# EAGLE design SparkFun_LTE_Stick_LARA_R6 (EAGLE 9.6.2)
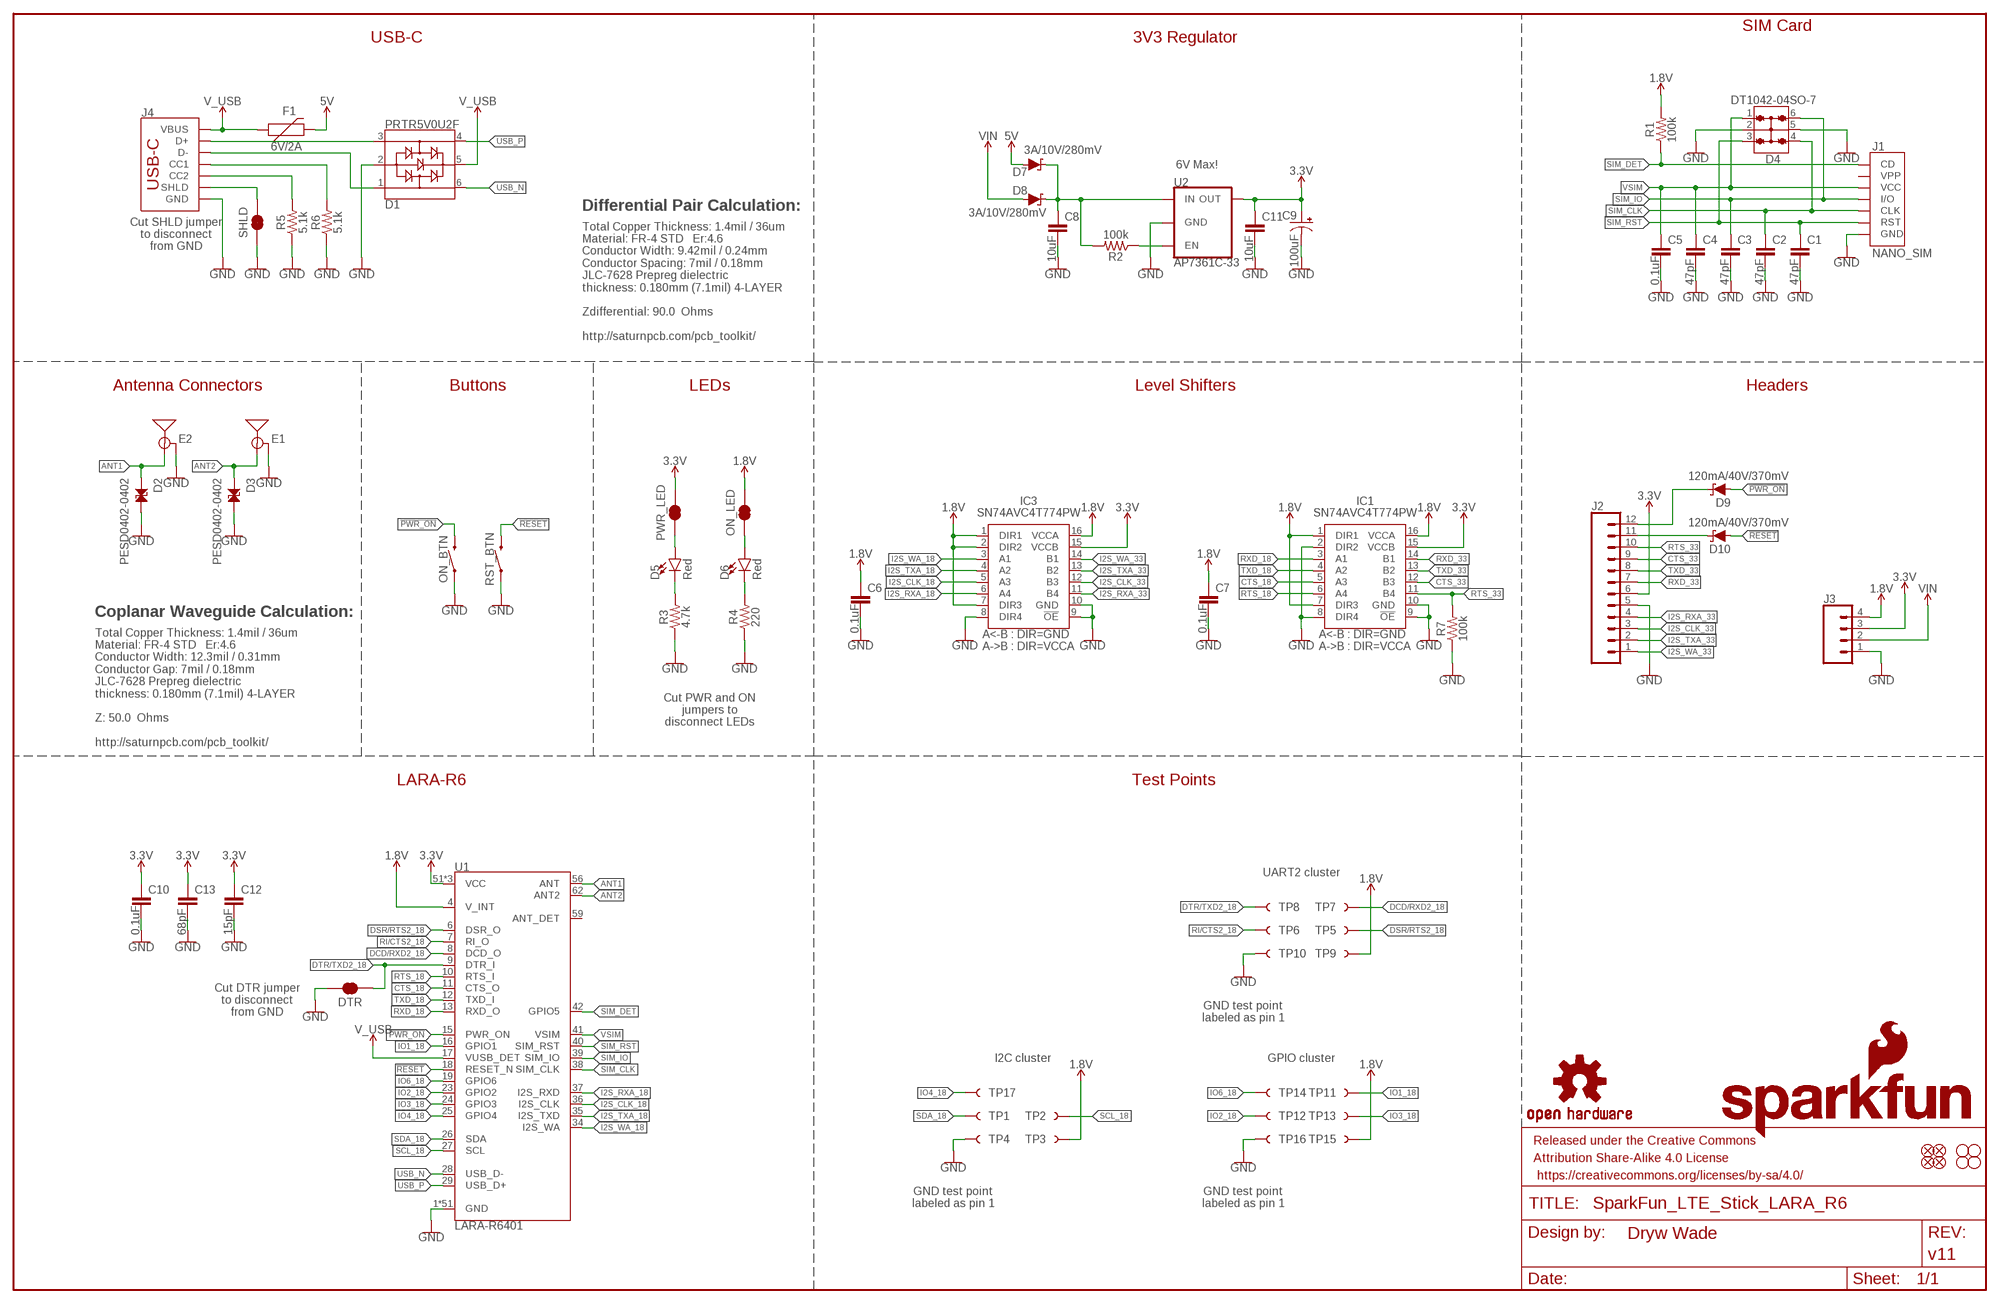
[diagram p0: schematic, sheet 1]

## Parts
C1  47pF  47PF-0603-50V-5%  [0603]
C2  47pF  47PF-0603-50V-5%  [0603]
C3  47pF  47PF-0603-50V-5%  [0603]
C4  47pF  47PF-0603-50V-5%  [0603]
C5  0.1uF  0.1UF-0603-25V-5%  [0603]
C6  0.1uF  0.1UF-0603-25V-5%  [0603]
C7  0.1uF  0.1UF-0603-25V-5%  [0603]
C8  10uF  10UF-0805-25V-10%  [0805]
C9  100uF  100UF-POLAR-25V-20%(ELEC)  [PANASONIC_D]
C10  0.1uF  0.1UF-0603-25V-5%  [0603]
C11  10uF  10UF-0805-25V-10%  [0805]
C12  15pF  15PF-0603-50V-5%  [0603]
C13  68pF  68PF-0603-50V-5%  [0603]
D1  PRTR5V0U2F  [SOT886]
D2  PESD0402-0402  [0402]
D3  PESD0402-0402  [0402]
D4  DT1042-04SO-7  TVS_DIODE_ARRAY_4_ESDA6V1BC6  [SOT23-6L]
D5  Red  LED-RED_0603-KB  [LED-0603]
D6  Red  LED-RED_0603-KB  [LED-0603]
D7  3A/10V/280mV  DIODE-SCHOTTKY-BAT60A  [SOD-323]
D8  3A/10V/280mV  DIODE-SCHOTTKY-BAT60A  [SOD-323]
D9  120mA/40V/370mV  DIODE-SCHOTTKY-RB751S40  [SOD-523]
D10  120mA/40V/370mV  DIODE-SCHOTTKY-RB751S40  [SOD-523]
DTR  JUMPER-SMT_2_NC_TRACE_SILK  [SMT-JUMPER_2_NC_TRACE_SILK]
E1  ANTENNA-SMA-GROUNDEDEDGE_SMA  [SMA-EDGE]
E2  ANTENNA-SMA-GROUNDEDEDGE_SMA  [SMA-EDGE]
F1  6V/2A  PPTC_6V2A  [1210]
FD1  FIDUCIAL1X2  [FIDUCIAL-1X2]
FD2  FIDUCIAL1X2  [FIDUCIAL-1X2]
FD3  FIDUCIAL1X2  [FIDUCIAL-1X2]
FD4  FIDUCIAL1X2  [FIDUCIAL-1X2]
FRAME1  FRAME-LEDGER  [CREATIVE_COMMONS]
H1  STAND-OFF  [STAND-OFF]
H2  STAND-OFF  [STAND-OFF]
H3  STAND-OFF  [STAND-OFF]
H4  STAND-OFF  [STAND-OFF]
IC1  SN74AVC4T774PW  [SOP65P640X120-16N]
IC3  SN74AVC4T774PW  [SOP65P640X120-16N]
J1  NANO_SIM  SIMHOLDER_WITH_CD-PUSHPUSH  [NANO_SIM_PP]
J2  CONN_12NO_SILK  [1X12_NO_SILK]
J3  CONN_041X04_NO_SILK_NO_POP  [1X04_NO_SILK]
J4  USB_C_4-LAYER_PADS  [USB-C-16P_4LAYER-PADS]
LOGO1  SFE_LOGO_NAME_FLAME.1_INCH  [SFE_LOGO_NAME_FLAME_.1]
LOGO2  OSHW-LOGOM  [OSHW-LOGO-M]
ON_BTN  MOMENTARY-SWITCH-SPST-SMD-4.6X2.8MM  [TACTILE_SWITCH_SMD_4.6X2.8MM]
ON_LED  JUMPER-SMT_2_NC_TRACE_SILK  [SMT-JUMPER_2_NC_TRACE_SILK]
PWR_LED  JUMPER-SMT_2_NC_TRACE_SILK  [SMT-JUMPER_2_NC_TRACE_SILK]
R1  100k  100KOHM-0603-1/10W-1%  [0603]
R2  100k  100KOHM-0603-1/10W-1%  [0603]
R3  4.7k  4.7KOHM-0603-1/10W-1%  [0603]
R4  220  220OHM-0603-1/10W-1%  [0603]
R5  5.1k  5.1KOHM5.1KOHM-0603-1/10W-1%  [0603]
R6  5.1k  5.1KOHM5.1KOHM-0603-1/10W-1%  [0603]
R7  100k  100KOHM-0603-1/10W-1%  [0603]
RST_BTN  MOMENTARY-SWITCH-SPST-SMD-4.6X2.8MM  [TACTILE_SWITCH_SMD_4.6X2.8MM]
SHLD  JUMPER-SMT_2_NC_TRACE_SILK  [SMT-JUMPER_2_NC_TRACE_SILK]
TP1  TEST-POINT3X5  [PAD.03X.05]
TP2  TEST-POINT3X5  [PAD.03X.05]
TP3  TEST-POINT3X5  [PAD.03X.05]
TP4  TEST-POINT3X5  [PAD.03X.05]
TP5  TEST-POINT3X5  [PAD.03X.05]
TP6  TEST-POINT3X5  [PAD.03X.05]
TP7  TEST-POINT3X5  [PAD.03X.05]
TP8  TEST-POINT3X5  [PAD.03X.05]
TP9  TEST-POINT3X5  [PAD.03X.05]
TP10  TEST-POINT3X5  [PAD.03X.05]
TP11  TEST-POINT3X5  [PAD.03X.05]
TP12  TEST-POINT3X5  [PAD.03X.05]
TP13  TEST-POINT3X5  [PAD.03X.05]
TP14  TEST-POINT3X5  [PAD.03X.05]
TP15  TEST-POINT3X5  [PAD.03X.05]
TP16  TEST-POINT3X5  [PAD.03X.05]
TP17  TEST-POINT3X5  [PAD.03X.05]
U1  LARA-R6401  LARA-R6_R6401_USA  [LARA-LGA]
U2  AP7361C-33  AP7361C-33FGEUDFN-8  [UDFN-8]

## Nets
1.8V: C6.1 C7.1 IC1.1(DIR1) IC1.7(DIR3) IC1.16(VCCA) IC3.1(DIR1) IC3.2(DIR2) IC3.7(DIR3) IC3.16(VCCA) J3.4 ON_LED.2 R1.2 TP3.1 TP9.1 TP15.1 U1.4(V_INT)
3.3V: C9.+ C10.1 C11.1 C12.1 C13.1 IC1.15(VCCB) IC3.15(VCCB) J2.6 J3.3 PWR_LED.2 U1.51(VCC) U1.52(VCC) U1.53(VCC) U2.1(OUT)
5V: D7.A F1.2
!PWR_ON!: D9.A ON_BTN.3 ON_BTN.4 U1.15(PWR_ON)
!RESET!: D10.A RST_BTN.3 RST_BTN.4 U1.18(RESET_N)
ANT1 [RF]: D2.1 E2.SIG(SIGNAL) U1.56(ANT)
ANT2 [RF]: D3.1 E1.SIG(SIGNAL) U1.62(ANT2)
CTS_18: IC1.5(A3) U1.11(CTS_O)
CTS_33: IC1.12(B3) J2.9
DCD/RXD2_18: TP7.1 U1.8(DCD_O)
DSR/RTS2_18: TP5.1 U1.6(DSR_O)
DTR/TXD2_18: DTR.2 TP8.1 U1.9(DTR_I)
EN: R2.1 U2.5(EN)
GND: C1.2 C2.2 C3.2 C4.2 C5.2 C6.2 C7.2 C8.2 C9.- C10.2 C11.2 C12.2 C13.2 D1.2 D2.2 D3.2 D4.2 D4.5 DTR.1 E1.GND@0(GND) E1.GND@1(GND) E1.GND@2(GND) E1.GND@3(GND) E2.GND@0(GND) E2.GND@1(GND) E2.GND@2(GND) E2.GND@3(GND) IC1.2(DIR2) IC1.8(DIR4) IC1.9(!OE) IC1.10(GND) IC3.8(DIR4) IC3.9(!OE) IC3.10(GND) J1.A1(GND) J1.A2(GND) J1.A3(GND) J1.A4(GND) J1.C5(GND) J2.5 J3.1 J4.GND J4.GND2(GND) ON_BTN.1 ON_BTN.2 R3.1 R4.1 R5.1 R6.1 R7.1 RST_BTN.1 RST_BTN.2 SHLD.1 TP4.1 TP10.1 TP16.1 U1.1(GND) U1.3(GND) U1.5(GND) U1.14(GND) U1.20(GND) U1.21(GND) U1.22(GND) U1.30(GND) U1.32(GND) U1.43(GND) U1.50(GND) U1.54(GND) U1.55(GND) U1.57(GND) U1.58(GND) U1.60(GND) U1.61(GND) U1.63(GND) U1.64(GND) U1.65(GND) U1.66(GND) U1.67(GND) U1.68(GND) U1.69(GND) U1.70(GND) U1.71(GND) U1.72(GND) U1.73(GND) U1.74(GND) U1.75(GND) U1.76(GND) U1.77(GND) U1.78(GND) U1.79(GND) U1.80(GND) U1.81(GND) U1.82(GND) U1.83(GND) U1.84(GND) U1.85(GND) U1.86(GND) U1.87(GND) U1.88(GND) U1.89(GND) U1.90(GND) U1.91(GND) U1.92(GND) U1.93(GND) U1.94(GND) U1.95(GND) U1.96(GND) U2.4(GND) U2.EP(GND)
I2S_CLK_18: IC3.5(A3) U1.36(I2S_CLK)
I2S_CLK_33: IC3.12(B3) J2.3
I2S_RXA_18: IC3.6(A4) U1.37(I2S_RXD)
I2S_RXA_33: IC3.11(B4) J2.4
I2S_TXA_18: IC3.4(A2) U1.35(I2S_TXD)
I2S_TXA_33: IC3.13(B2) J2.2
I2S_WA_18: IC3.3(A1) U1.34(I2S_WA)
I2S_WA_33: IC3.14(B1) J2.1
IO1_18: TP11.1 U1.16(GPIO1)
IO2_18: TP12.1 U1.23(GPIO2)
IO3_18: TP13.1 U1.24(GPIO3)
IO4_18: TP17.1 U1.25(GPIO4)
IO6_18: TP14.1 U1.19(GPIO6)
N$1: D5.C R3.2
N$2: D5.A PWR_LED.1
N$3: D6.A ON_LED.1
N$4: D6.C R4.2
N$5: D10.C J2.11
N$6: D9.C J2.12
N$7: C8.1 D7.C D8.C R2.2 U2.8(IN)
N$8: J4.B5(CC2) R5.2
N$9: J4.A5(CC1) R6.2
N$10: D1.3 J4.A6(D+) J4.B6(D+)
N$11: D1.1 J4.A7(D-) J4.B7(D-)
RI/CTS2_18: TP6.1 U1.7(RI_O)
RTS_18: IC1.6(A4) U1.10(RTS_I)
RTS_33: IC1.11(B4) J2.10 R7.2
RXD_18: IC1.3(A1) U1.13(RXD_O)
RXD_33: IC1.14(B1) J2.7
SCL_18: TP2.1 U1.27(SCL)
SDA_18: TP1.1 U1.26(SDA)
SHLD: J4.SHLD1(SHLD) J4.SHLD2(SHLD) J4.SHLD3(SHLD) J4.SHLD4(SHLD) SHLD.2
SIM_CLK: C2.1 D4.4 J1.C3(CLK) U1.38(SIM_CLK)
SIM_DET: J1.CD R1.1 U1.42(GPIO5)
SIM_IO: C3.1 D4.6 J1.C7(I/O) U1.39(SIM_IO)
SIM_RST: C1.1 D4.3 J1.C2(RST) U1.40(SIM_RST)
TXD_18: IC1.4(A2) U1.12(TXD_I)
TXD_33: IC1.13(B2) J2.8
USB_N [USB]: D1.6 U1.28(USB_D-)
USB_P [USB]: D1.4 U1.29(USB_D+)
V_USB: D1.5 F1.1 J4.VBUS1(VBUS) J4.VBUS2(VBUS) U1.17(VUSB_DET)
VIN: D8.A J3.2
VSIM: C4.1 C5.1 D4.1 J1.C1(VCC) U1.41(VSIM)
Unconnected: J1.C6(VPP) U1.59(ANT_DET)

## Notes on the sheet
- SIM Card
- USB-C | 3V3 Regulator
- 6V Max!
- Differential Pair Calculation:
- Total Copper Thickness: 1.4mil / 36um
  Material: FR-4 STD   Er:4.6
  Conductor Width: 9.42mil / 0.24mm
  Conductor Spacing: 7mil / 0.18mm
  JLC-7628 Prepreg dielectric
  thickness: 0.180mm (7.1mil) 4-LAYER
  
  Zdifferential: 90.0  Ohms
  
  http://saturnpcb.com/pcb_toolkit/
- Cut SHLD jumper
  to disconnect
  from GND
- Antenna Connectors | Buttons | LEDs | Level Shifters | Headers
- Coplanar Waveguide Calculation:
- Total Copper Thickness: 1.4mil / 36um
  Material: FR-4 STD   Er:4.6
  Conductor Width: 12.3mil / 0.31mm
  Conductor Gap: 7mil / 0.18mm
  JLC-7628 Prepreg dielectric
  thickness: 0.180mm (7.1mil) 4-LAYER
  
  Z: 50.0  Ohms
  
  http://saturnpcb.com/pcb_toolkit/
- Cut PWR and ON
  jumpers to
  disconnect LEDs
- LARA-R6 | Test Points
- UART2 cluster
- Cut DTR jumper
  to disconnect
  from GND
- GND test point
  labeled as pin 1
- I2C cluster | GPIO cluster
- GND test point
  labeled as pin 1
- GND test point
  labeled as pin 1

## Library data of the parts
C1-C4 = SparkFun-Capacitors:47PF: 47pF ceramic capacitors; PROD_ID: CAP-08913
C5-C7 C10 = SparkFun-Capacitors:0.1UF: 0.1µF ceramic capacitors; PROD_ID: CAP-08604
C8 C11 = SparkFun-Capacitors:10UF: 10.0µF ceramic capacitors; PROD_ID: CAP-14259
C9 = SparkFun-Capacitors:100UF-POLAR: 100µF polarized capacitors; PROD_ID: CAP-12547
C12 = SparkFun-Capacitors:15PF: 15pF ceramic capacitors; PROD_ID: CAP-07881
C13 = SparkFun-Capacitors:68PF: 68pF ceramic capacitors; PROD_ID: CAP-14092
D1 = SparkFun-IC-Power:PRTR5V0U2: A small ESD protection device. Most commonly used on USB D+/D- signals to protect large, expensive, or especially sensitive USB enabled devices.; PROD_ID: DIO-14084
D2 D3 = SparkFun-DiscreteSemi:PESD0402: ESD protection diode; DIGIKEY_PART: PESD0402-140CT-ND; MOUSE_PART: 650-PESD0402-140; PROD_ID: DIO-15359
D4 = SparkFun-DiscreteSemi:TVS_DIODE_ARRAY_4; PROD_ID: DIO-14095
D5 D6 = SparkFun-LED:LED-RED: Red SMD LED; PROD_ID: DIO-17976
D7 D8 = SparkFun-DiscreteSemi:DIODE-SCHOTTKY: Schottky diode; PROD_ID: DIO-14072
D9 D10 = SparkFun-DiscreteSemi:DIODE-SCHOTTKY: Schottky diode; PROD_ID: DIO-11018
DTR ON_LED PWR_LED SHLD = SparkFun-Jumpers:JUMPER-SMT_2_NC_TRACE: Normally closed trace jumper
E1 E2 = SparkFun-RF:ANTENNA-SMA-GROUNDED: SMA Antenna Connector w/ Ground; PROD_ID: CONN-19593
F1 = SparkFun-Fuses:PPTC: Resettable Fuse PPTC; PROD_ID: RES-14313
FD1-FD4 = SparkFun-Aesthetics:FIDUCIAL: Fiducial Alignment Points
FRAME1 = SparkFun-Aesthetics:FRAME-LEDGER: Schematic Frame - Ledger; DESIGNER: Dryw Wade; REV: v11
H1-H4 = SparkFun-Hardware:STAND-OFF: Stand Off
IC1 IC3 = SparkFun-IC-Comms:SN74AVC4T774PW: Texas Instruments,SN74AVC4T774PW,IC, Texas Instruments SN74AVC4T774PW, Dual, Bus Transceiver, 4-Bit Non-Inverting 3-State, 1.2 3.6 V, 16-Pin TSSOP Source: Datasheet; PROD_ID: IC-15360
J1 = SparkFun-Connectors:SIMHOLDER_WITH_CD: SIM Cellular Card Socket SMT 6 pin standard connection. SparkFun Products: SIM Socket SparkFun Cellular Shield - MG2639 SparkFun SIM Card Socket Breakout; PROD_ID: CONN-16272
J2 = SparkFun-Connectors:CONN_12: Multi connection point. Often used as Generic Header-pin footprint for 0.1 inch spaced/style header connections On any of the 0.1 inch spaced packages, you can populate with these: Break Away Headers - Straight (PRT-00116) Break Away Male Headers - Right Angle (PRT-00553) Female Headers (PRT-00115)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
J3 = SparkFun-Connectors:CONN_04: Multi connection point. Often used as Generic Header-pin footprint for 0.1 inch spaced/style header connections On any of the 0.1 inch spaced packages, you can populate with these: Break Away Headers - Straight (PRT-00116) Break Away Male Headers - Right Angle (PRT-00553) Female Headers (PRT-00115)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
J4 = SparkFun-Connectors:USB_C: USB Type C 16Pin Connector Super Speed pins not available on the 16-pin purely SMD connector so this part is best for USB 2.0 implementations. D1 and D2 are tied together enabling D+/- no matter which way the cable is plugged into the connector. The two channel configuration pins (CC1/2) are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; PROD_ID: CONN-14122
LOGO1 = SparkFun-Aesthetics:SFE_LOGO_NAME_FLAME: SparkFun Font Logo w/ Flame
LOGO2 = SparkFun-Aesthetics:OSHW-LOGO: Open-Source Hardware (OSHW) Logo
ON_BTN RST_BTN = SparkFun-Switches:MOMENTARY-SWITCH-SPST: Momentary Switch (Pushbutton) - SPST; PROD_ID: SWCH-15606
R1 R2 R7 = SparkFun-Resistors:100KOHM: 100kΩ resistor; PROD_ID: RES-07828
R3 = SparkFun-Resistors:4.7KOHM: 4.7kΩ resistor; PROD_ID: RES-07857
R4 = SparkFun-Resistors:220OHM: 220Ω resistor; PROD_ID: RES-07861
R5 R6 = SparkFun-Resistors:5.1KOHM; PROD_ID: RES-12083
TP1-TP17 = SparkFun-Connectors:TEST-POINT: SparkFun Test Points
U1 = SparkFun-RF:LARA-R6: u-blox LARA-R6 single or multi-mode LTE Cat 1 modules; PROD_ID: IC-16756
U2 = SparkFun-IC-Power:AP7361C-33FGE: AP7361C 3.3V LDO Regulator; PROD_ID: VREG-14094

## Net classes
1 USB: width 0.239 mm, clearance 0.178 mm
2 RF: width 0.312 mm, clearance 0.178 mm to class 0

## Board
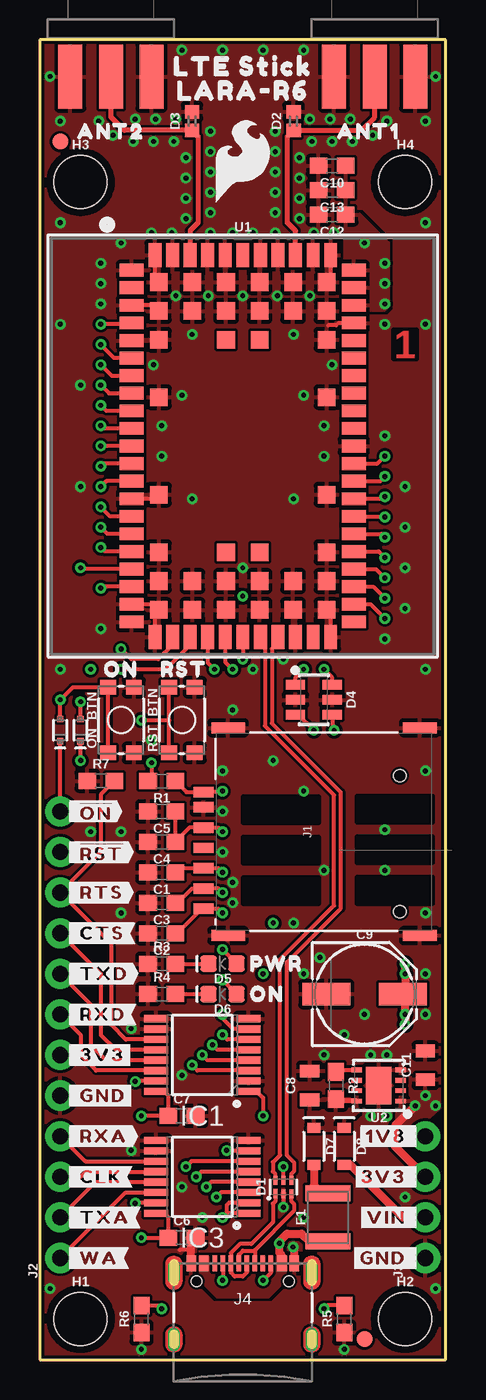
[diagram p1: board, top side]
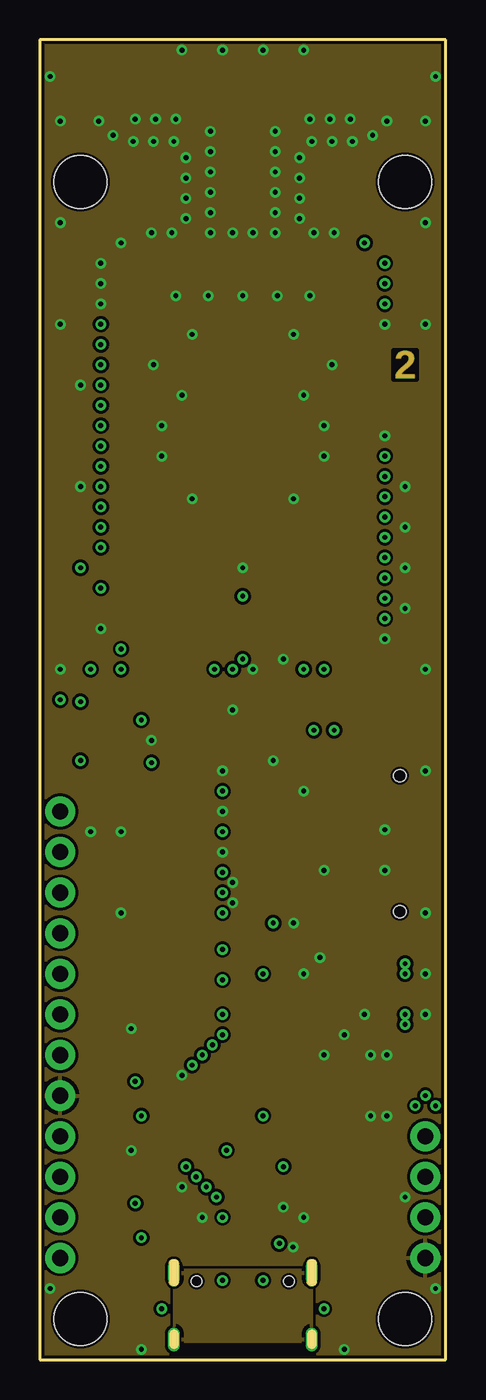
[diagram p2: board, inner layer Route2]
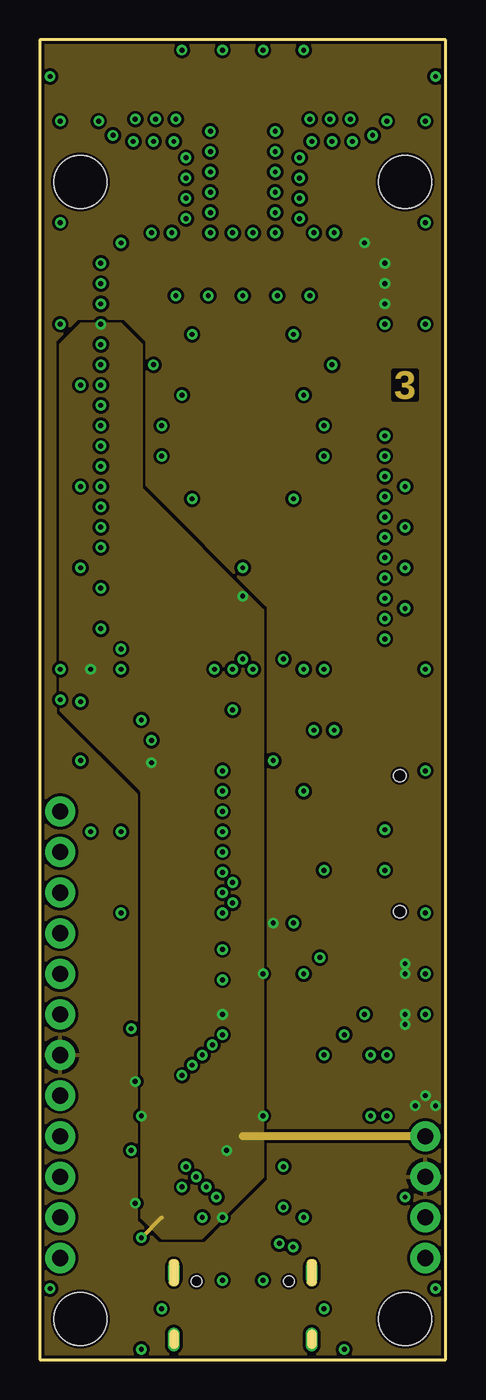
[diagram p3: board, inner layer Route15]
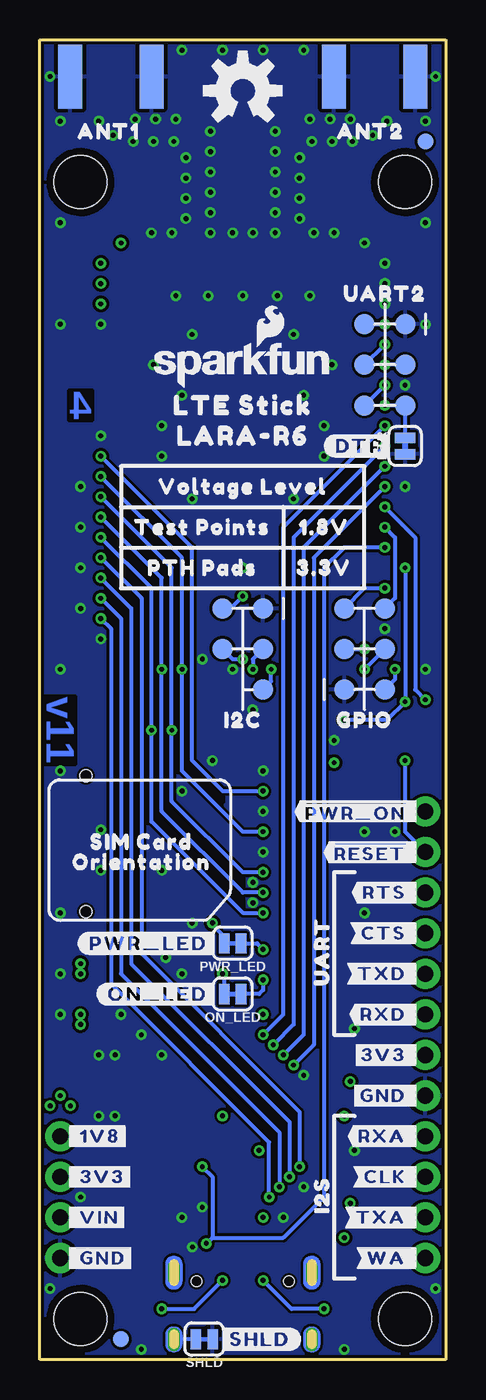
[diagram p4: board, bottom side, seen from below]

Size 25.4 x 82.55 mm. Coordinates in mm from the lower left corner, seen from the top.
Outline: 0,0 25.4,0 25.4,82.55 0,82.55 0,0
Copper layers (1+2*15+16): Top 0.035559375mm / dielectric 0.47751875mm / Route2 0.035559375mm / dielectric 0.47751875mm / Route15 0.035559375mm / dielectric 0.47751875mm / Bottom 0.035559375mm
Design rules "SparkFun-4-Layer-General-JLCPCB": minimum track width 7mil, minimum drill 12mil, track to track 7mil, track to pad 7mil, pad to pad 7mil, via to via 7mil, smd to smd 7mil, copper to edge 7mil, drill to drill 7mil, minimum pad ring 7mil, minimum via ring 7mil, stop-mask expansion 3mil, vias tented up to drill 25mil, thermal gap 10mil
tRestrict: area 7.1,23.6 to 7.2,24; area 7.1,13.3 to 7.5,13.5; area 7.1,21 to 7.5,21.1
bRestrict: area 12.7,28.4 to 12.8,28.7; area 12.7,29.7 to 12.8,30; area 14,34.9 to 14.1,35.2

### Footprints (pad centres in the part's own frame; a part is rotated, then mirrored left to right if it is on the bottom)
0603 = smd 1.1 x 1: 1 -0.85,0; 2 0.85,0
0805 = smd 0.8 x 1.2: 1 -0.9,0; 2 0.9,0
PANASONIC_D = smd 3 x 1.4: + 2.4,0; - -2.4,0
SOT886 = smd 0.61 x 0.25: 1 -0.405,0.5 | smd 0.56 x 0.25: 2 -0.43,0; 3 -0.43,-0.5; 4 0.43,-0.5; 5 0.43,0; 6 0.43,0.5
0402 = smd 0.85 x 0.9: 1 -0.58,0; 2 0.58,0
SOT23-6L = smd 0.6 x 1.2: 1 -0.95,-1.15; 2 0,-1.15; 3 0.95,-1.15; 4 0.95,1.15; 5 0,1.15; 6 -0.95,1.15
LED-0603 = smd 1 x 1: A -0.877,0; C 0.877,0
SOD-323 = smd 0.63 x 0.83: A 1.15,0; C -1.15,0
SOD-523 = smd 0.4 x 0.4: A -0.7,0; C 0.7,0
SMT-JUMPER_2_NC_TRACE_SILK = smd 0.66 x 1.27: 1 -0.521,0; 2 0.521,0
SMA-EDGE = smd 1.5 x 4: GND@0 -2.54,0; GND@1 2.54,0; SIG 0,0 | smd 1.5 x 4 bottom: GND@2 -2.54,0; GND@3 2.54,0
1210 = smd 1 x 2.8: 1 -1.5,0; 2 1.5,0
FIDUCIAL-1X2 = smd 1 x 1: 1 0,0
STAND-OFF = hole 3.302: 0,0
SOP65P640X120-16N = smd 1.5 x 0.45: 1 -2.9,2.275; 2 -2.9,1.625; 3 -2.9,0.975; 4 -2.9,0.325; 5 -2.9,-0.325; 6 -2.9,-0.975; 7 -2.9,-1.625; 8 -2.9,-2.275; 9 2.9,-2.275; 10 2.9,-1.625; 11 2.9,-0.975; 12 2.9,-0.325; 13 2.9,0.325; 14 2.9,0.975; 15 2.9,1.625; 16 2.9,2.275
NANO_SIM_PP = smd 0.7 x 2.1: A1 6.495,6; A2 -6.495,6; A3 -6.495,-6; A4 6.495,-6 | smd 0.65 x 1.23: C1 0.255,7.535; C2 -2.285,7.535; C3 -4.825,7.535; C5 1.525,7.535; C6 -1.015,7.535; C7 -3.555,7.535; CD 2.475,7.535 | hole 0.75: 3.505,-4.75; -4.995,-4.75
1X12_NO_SILK = drill 1.016 pad 1.88: 1 0,0; 2 2.54,0; 3 5.08,0; 4 7.62,0; 5 10.16,0; 6 12.7,0; 7 15.24,0; 8 17.78,0; 9 20.32,0; 10 22.86,0; 11 25.4,0; 12 27.94,0
1X04_NO_SILK = drill 1.016 pad 1.88: 1 0,0; 2 2.54,0; 3 5.08,0; 4 7.62,0
USB-C-16P_4LAYER-PADS = smd 0.3 x 1: A5 -1.25,-0.34; A6 -0.25,-0.34; A7 0.25,-0.34; A8 1.25,-0.34; B5 1.75,-0.34; B6 0.75,-0.34; B7 -0.75,-0.34; B8 -1.75,-0.34 | smd 0.6 x 1: GND -3.225,-0.34; GND2 3.225,-0.34; VBUS1 -2.45,-0.34; VBUS2 2.45,-0.34 | drill 0.4 pad 0.6 long: SHLD1 -4.318,-0.915; SHLD2 4.318,-0.915; SHLD3 -4.318,-5.095; SHLD4 4.318,-5.095 | hole 0.65: -2.89,-1.445; 2.89,-1.445
TACTILE_SWITCH_SMD_4.6X2.8MM = smd 0.9 x 1: 1 -2.05,-0.8; 2 2.05,-0.8; 3 2.05,0.8; 4 -2.05,0.8
PAD.03X.05 = smd 1.27 x 1.27: 1 0,0
LARA-LGA = smd 0.8 x 1.5: 1 -11,-6.95; 2 -9.9,-6.95; 3 -8.8,-6.95; 4 -7.7,-6.95; 5 -6.6,-6.95; 6 -5.5,-6.95; 7 -4.4,-6.95; 8 -3.3,-6.95; 9 -2.2,-6.95; 10 -1.1,-6.95; 11 0,-6.95; 12 1.1,-6.95; 13 2.2,-6.95; 14 3.3,-6.95; 15 4.4,-6.95; 16 5.5,-6.95; 17 6.6,-6.95; 18 7.7,-6.95; 19 8.8,-6.95; 20 9.9,-6.95; 21 11,-6.95; 33 11,6.95; 34 9.9,6.95; 35 8.8,6.95; 36 7.7,6.95; 37 6.6,6.95; 38 5.5,6.95; 39 4.4,6.95; 40 3.3,6.95; 41 2.2,6.95; 42 1.1,6.95; 43 0,6.95; 44 -1.1,6.95; 45 -2.2,6.95; 46 -3.3,6.95; 47 -4.4,6.95; 48 -5.5,6.95; 49 -6.6,6.95; 50 -7.7,6.95; 51 -8.8,6.95; 52 -9.9,6.95; 53 -11,6.95 | smd 1.5 x 0.8: 22 11.95,-5.5; 23 11.95,-4.4; 24 11.95,-3.3; 25 11.95,-2.2; 26 11.95,-1.1; 27 11.95,0; 28 11.95,1.1; 29 11.95,2.2; 30 11.95,3.3; 31 11.95,4.4; 32 11.95,5.5; 54 -11.95,5.5; 55 -11.95,4.4; 56 -11.95,3.3; 57 -11.95,2.2; 58 -11.95,1.1; 59 -11.95,0; 60 -11.95,-1.1; 61 -11.95,-2.2; 62 -11.95,-3.3; 63 -11.95,-4.4; 64 -11.95,-5.5 | smd 1.1 x 1.1: 65 -10.25,-5.25; 66 -10.25,-3.15; 67 -10.25,-1.05; 68 -10.25,1.05; 69 -10.25,3.15; 70 -10.25,5.25; 71 -8.45,-5.25; 72 -8.45,-3.15; 73 -8.45,-1.05; 74 -8.45,1.05; 75 -8.45,3.15; 76 -8.45,5.25; 77 -6.65,-5.25; 78 -6.65,5.25; 79 -3.05,-5.25; 80 -3.05,5.25; 81 3.05,-5.25; 82 3.05,5.25; 83 6.65,-5.25; 84 6.65,5.25; 85 8.45,-5.25; 86 8.45,-3.15; 87 8.45,-1.05; 88 8.45,1.05; 89 8.45,3.15; 90 8.45,5.25; 91 10.25,-5.25; 92 10.25,-3.15; 93 10.25,-1.05; 94 10.25,1.05; 95 10.25,3.15; 96 10.25,5.25; 97 -6.65,-1.05; 98 -6.65,1.05; 99 6.65,-1.05; 100 6.65,1.05
UDFN-8 = smd 0.3 x 0.65: 1 -0.975,-1.375; 2 -0.325,-1.375; 3 0.325,-1.375; 4 0.975,-1.375; 5 0.975,1.375; 6 0.325,1.375; 7 -0.325,1.375; 8 -0.975,1.375 | smd 2.35 x 1.6: EP 0,0

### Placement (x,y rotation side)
C1  7.62,30.48 180 top
C2  7.62,26.67 180 top
C3  7.62,28.57 180 top
C4  7.62,32.38 180 top
C5  7.62,34.29 180 top
C6  8.89,7.62 0 top
C7  8.89,15.24 0 top
C8  16.89,17.14 90 top
C9  20.32,22.86 0 top
C10  18.29,74.68 180 top
C11  24.13,18.41 90 top
C12  18.29,71.63 180 top
C13  18.29,73.15 180 top
D1  15.24,10.79 90 top
D2  15.88,77.47 90 top
D3  9.53,77.47 90 top
D4  17.14,41.27 270 top
D5  11.43,24.77 180 top
D6  11.43,22.86 180 top
D7  17.14,13.34 270 top
D8  19.05,13.34 270 top
D9  1.27,39.37 270 top
D10  2.54,39.37 270 top
DTR  2.54,57.15 90 bottom
E1  4.45,80.26 0 top
E2  20.95,80.26 0 top
F1  18.03,8.89 90 top
FD1  1.27,76.2 0 top
FD2  1.27,76.2 0 bottom
FD3  20.32,1.27 0 top
FD4  20.32,1.27 0 bottom
FRAME1  not placed on the board
H1  2.54,2.54 0 top
H2  22.86,2.54 0 top
H3  2.54,73.66 0 top
H4  22.86,73.66 0 top
IC1  10.16,19.05 180 top
IC3  10.16,11.43 180 top
J1  17.78,33.02 90 top
J2  1.27,6.35 90 top
J3  24.13,6.35 90 top
J4  12.7,6.35 0 top
LOGO1  12.7,62.23 0 bottom
LOGO2  12.7,79.38 0 bottom
ON_BTN  5.08,40.01 90 top
ON_LED  13.34,22.86 180 bottom
PWR_LED  13.34,26.04 180 bottom
R1  7.62,36.2 180 top
R2  18.54,17.14 270 top
R3  7.62,24.77 0 top
R4  7.62,22.86 0 top
R5  19.05,2.54 90 top
R6  6.35,2.54 90 top
R7  3.81,36.2 0 top
RST_BTN  8.89,40.01 90 top
SHLD  15.11,1.27 180 bottom
TP1  11.43,44.45 180 bottom
TP2  13.97,44.45 180 bottom
TP3  13.97,46.99 180 bottom
TP4  11.43,46.99 180 bottom
TP5  5.08,62.23 180 bottom
TP6  2.54,62.23 180 bottom
TP7  5.08,59.69 180 bottom
TP8  2.54,59.69 180 bottom
TP9  5.08,64.77 180 bottom
TP10  2.54,64.77 180 bottom
TP11  3.81,46.99 0 bottom
TP12  6.35,44.45 0 bottom
TP13  3.81,44.45 0 bottom
TP14  6.35,46.99 0 bottom
TP15  3.81,41.91 0 bottom
TP16  6.35,41.91 0 bottom
TP17  11.43,41.91 0 bottom
U1  12.7,57.15 270 top
U2  21.21,17.14 90 top
U$1  [LTE_STICK0]  12.7,80.9 0 top
U$2  [SFE_LOGO_FLAME_.2]  12.7,74.93 0 top
U$3  [#_3V3#0]  1.52,19.05 0 top
U$4  [#_GND#0]  1.52,16.51 0 top
U$5  [#_GND#0]  23.88,6.35 0 bottom
U$6  [#SHLD#0]  14.22,1.27 0 bottom
U$7  [#GND_#0]  23.88,6.35 0 top
U$8  [#GND_#0]  1.52,16.51 0 bottom
U$9  [#3V3_#0]  1.52,19.05 0 bottom
U$10  [#DTR#0]  3.17,57.15 0 bottom
U$11  [#VIN_#0]  23.88,8.89 0 top
U$12  [#3V3_#0]  23.88,11.43 0 top
U$13  [#1V8_#0]  23.88,13.97 0 top
U$14  [#_1V8#0]  23.88,13.97 0 bottom
U$15  [#_3V3#0]  23.88,11.43 0 bottom
U$16  [#_VIN#0]  23.88,8.89 0 bottom
U$17  [#_CTS#0]  1.52,26.67 0 top
U$18  [#_RTS#0]  1.52,29.21 0 top
U$19  [#RXD_#0]  1.52,21.59 0 bottom
U$20  [#TXD_#0]  1.52,24.13 0 bottom
U$21  [#_CLK#0]  1.52,11.43 0 top
U$22  [#_WA#0]  1.52,6.35 0 top
U$23  [#RXA_#0]  1.52,13.97 0 bottom
U$24  [#TXA_#0]  1.52,8.89 0 bottom
U$25  [LTE_STICK0]  12.7,59.69 0 bottom
U$26  [SIM_CARD0]  19.05,32.38 0 bottom
U$27  [VOLTAGE_LEVEL0]  12.7,54.61 0 bottom
U$28  [PWR0]  12.45,24.77 0 top
U$29  [ANT10]  20.57,76.83 0 top
U$30  [TEST_POINTS0]  15.24,52.07 0 bottom
U$31  [LARA#R60]  12.7,79.38 0 top
U$32  [#_RXA#0]  1.52,13.97 0 top
U$33  [#_#RST##0]  1.52,31.75 0 top
U$34  [PTH_PADS0]  15.24,49.53 0 bottom
U$35  [LARA#R60]  12.7,57.78 0 bottom
U$36  [ANT10]  21.08,76.83 0 bottom
U$37  [ON0]  3.3,43.18 0 top
U$38  [##PWR_ON#_#0]  1.52,34.29 0 bottom
U$39  [ON0]  12.45,22.86 0 top
U$40  [#_TXA#0]  1.52,8.89 0 top
U$41  [#_TXD#0]  1.52,24.13 0 top
U$42  [#_RXD#0]  1.52,21.59 0 top
U$43  [#CLK_#0]  1.52,11.43 0 bottom
U$44  [#WA_#0]  1.52,6.35 0 bottom
U$45  [#RTS_#0]  1.52,29.21 0 bottom
U$46  [#CTS_#0]  1.52,26.67 0 bottom
U$47  [##RESET#_#0]  1.52,31.75 0 bottom
U$48  [UART0]  7.75,25.53 90 bottom
U$49  [I2S0]  7.75,10.29 90 bottom
U$50  [1#8V0]  7.62,52.07 0 bottom
U$51  [ORIENTATION0]  19.05,31.11 0 bottom
U$52  [RST0]  9.02,43.18 0 top
U$53  [#ON_LED#0]  14.22,22.86 0 bottom
U$54  [3#3V0]  7.62,49.53 0 bottom
U$55  [ORDERING_INSTRUCTIONS]  not placed on the board
U$56  [UART20]  3.81,66.67 0 bottom
U$57  [GPIO0]  5.08,40.01 0 bottom
U$58  [I2C0]  12.7,40.01 0 bottom
U$59  [#_#ON##0]  1.52,34.29 0 top
U$60  [#PWR_LED#0]  14.22,26.04 0 bottom
U$61  [ANT20]  4.7,76.83 0 bottom
U$62  [ANT20]  4.45,76.83 0 top

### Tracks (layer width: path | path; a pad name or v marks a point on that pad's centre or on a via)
1.8V  (via drill 0.3)
  Top 0.254: U1.4 5.67,64.77 v3.81,64.77 | v6.35,15.24 C7.1 8.04,16.51 7.78,16.77 IC1.16 | v6.35,7.62 C6.1 8.04,8.89 7.78,9.15 IC3.16 | IC3.7 11.71,13.05 v11.68,13.08 | IC1.7 12.09,20.68 11.43,21.34 v11.43,21.59 | IC3.1 11.7,9.15 | 11.7,9.15 v11.43,8.89 | IC1.1 13.57,16.77 13.97,16.37 v13.97,15.24 | v6.99,37.34 6.99,36.41 R1.2 | IC3.2 11.84,9.8 11.7,9.66 11.7,9.15
  Route15 0.254: v6.35,7.62 7.62,8.89
  Route15 0.508: J3.4 12.7,13.97
  Bottom 0.254: TP9.1 v3.81,64.77 | v3.17,43.18 3.17,42.55 TP15.1 | TP3.1 13.46,46.99 v12.7,47.75 | ON_LED.2 13.86,24.02 v13.97,24.13
  pour Route15 (isolate 0.178): 5.08,64.77 2.54,64.77 1.27,63.5 1.27,40.64 6.35,35.56 6.35,8.89 7.62,7.62 10.16,7.62 13.97,11.43 13.97,46.86 6.35,54.48 6.35,63.5
3.3V  (via drill 0.3)
  Top 0.254: IC1.15 6,17.43 v5.97,17.4 | IC3.15 6,9.8 v5.97,9.78
  Top 0.508: v22.86,20.95 v22.86,21.59 22.86,22.72 C9.+ 22.86,23 v22.86,24.13 v22.86,24.77 | J3.3 22.23,13.34 22.23,14.61 v23.5,15.88
  Bottom 0.254: v14.61,27.3 14.61,27.18 13.86,26.43 PWR_LED.2
  other vias: 21.59,66.04 21.59,67.31 21.59,68.58 20.32,69.85 24.13,16.51 24.77,15.88
  pour Route15 (isolate 0.178, rank 2): 25.4,0 0,0 0,82.55 25.4,82.55
  pour Top (isolate 0.178): 22.35,14.73 22.35,17.65 25.02,17.65 25.02,15.75 24,14.73
  pour Top (isolate 0.178): 19.05,65.66 21.59,65.66 21.84,65.91 21.84,69.85 19.56,72.14 19.56,75.06 18.67,75.06 18.67,71.12 19.05,70.74
5V
  Top 0.508: D7.A 17.14,10.9 17.65,10.39 F1.2
!PWR_ON!  (via drill 0.3)
  Top 0.254: U1.15 4.4,52.75 v3.81,53.34 | D9.A v1.27,41.27 2.05,42.05 ON_BTN.3 ON_BTN.4
  Bottom 0.254: v3.81,53.34 1.91,51.44 1.91,41.91 v1.27,41.27
!RESET!  (via drill 0.3)
  Top 0.254: U1.18 2.62,49.45 v2.54,49.53 | D10.A v2.54,41.15 | RST_BTN.4 8.09,40.01 | 8.09,40.01 RST_BTN.3 | v6.35,40.01 8.09,40.01
  Bottom 0.254: v2.54,49.53 v2.54,41.15 3.68,40.01 v6.35,40.01
ANT1
  Top 0.312: U1.56 16,70.61 15.49,71.12 15.49,76.51 D2.1 20.12,76.89 20.95,77.72 E2.SIG
ANT2
  Top 0.312: U1.62 9.4,70.62 9.91,71.13 9.91,76.51 D3.1 5.28,76.89 4.45,77.72 E1.SIG
CTS_18  (via drill 0.3)
  Top 0.254: U1.11 v3.81,57.15 | IC1.5 11.11,19.38 v10.79,19.68
  Bottom 0.254: v3.81,57.15 9.53,51.44 9.53,20.95 v10.79,19.68
CTS_33
  Top 0.254: IC1.12 4.75,19.38 3.81,20.32 3.81,24.13 J2.9
DCD/RXD2_18  (via drill 0.3)
  Top 0.254: v3.81,60.96 4.32,60.45 U1.8
  Bottom 0.254: TP7.1 v3.81,60.96
DSR/RTS2_18  (via drill 0.3)
  Top 0.254: v3.81,63.5 4.66,62.65 U1.6
  Bottom 0.254: TP5.1 v3.81,63.5
DTR/TXD2_18  (via drill 0.3)
  Top 0.254: v3.81,59.69 4.15,59.35 U1.9
  Bottom 0.254: v3.81,59.69 TP8.1 DTR.2
EN
  Top 0.254: R2.1 18.67,18.12 U2.5
GND  (via drill 0.3)
  Top 0.239: D1.2 v15.24,9.53
  Top 0.254: 9.49,6.86 8.76,6.86 | U1.14 7.2,53.85 U1.81 | U1.71 7.1,65.95 U1.3 | U1.65 7.2,67.65 U1.64 | U1.70 18.2,67.65 U1.54 | U1.50 18.69,64.85 18.54,64.71 18.03,64.71 | U1.22 7.2,46.65 U1.91 7.1,47.25 U1.20 | U1.32 18.2,46.65 U1.96
  Top 0.508: J4.GND2 15.93,6.96 v15.85,7.04 | J4.GND 9.47,7.36 C6.2
  other vias: 6.35,0.64 19.05,0.64 11.43,34.29 13.34,43.18 15.24,43.81 17.78,30.61 14.73,71.75 14.73,73.03 14.73,74.3 14.73,75.56 16.89,77.6 18.16,77.6 19.43,77.6 16.26,71.37 16.26,72.64 16.26,73.91 16.26,75.18 17.02,76.2 18.29,76.2 19.56,76.2 17.14,70.48 18.41,70.48 14.73,70.48 13.34,70.48 12.06,70.48 10.67,70.48 10.67,71.75 10.67,73.03 10.67,74.3 10.67,75.56 10.67,76.83 8.51,77.6 7.24,77.6 5.97,77.6 9.14,71.37 9.14,72.64 9.14,73.91 9.14,75.18 8.38,76.2 7.11,76.2 5.84,76.2 3.68,77.47 8.26,70.48 6.99,70.48 21.72,77.47 20.83,76.58 14.73,76.83 4.57,76.58 3.81,67.31 3.81,66.04 3.81,68.58 5.08,69.85 21.59,57.78 21.59,64.77 12.7,49.53 3.81,45.72 21.59,45.09 8.89,81.92 16.51,81.92 11.43,81.92 13.97,81.92 24.13,77.47 24.13,71.12 1.27,71.12 1.27,77.47 1.27,64.77 24.13,64.77 0.64,80.26 24.77,80.26 0.64,4.45 24.77,4.45 16.51,8.89 10.16,8.89 8.89,17.78 8.89,10.79 5.71,20.7 5.71,13.08 5.08,27.94 5.08,33.02 1.27,43.18 12.06,40.64 11.43,36.83 24.13,21.59 17.78,19.05 16.51,24.13 17.53,25.15 24.13,24.13 24.13,27.94 24.13,36.83 24.13,43.18 14.61,37.47 11.43,31.75 22.86,49.53 22.86,54.61 22.86,52.07 22.86,46.99 2.54,54.61 2.54,60.96 7.11,62.23 18.29,62.23 17.78,58.42 7.62,58.42 9.53,53.85 15.88,53.85 12.7,66.55 8.51,66.55 16.89,66.55 10.54,66.55 14.86,66.55 15.88,64.14 9.53,64.14 8.89,60.33 16.51,60.33 7.62,56.52 17.78,56.52 22.86,10.16 16.51,35.56 21.59,30.61 21.59,33.15 3.17,33.02 6.99,38.73 20.7,19.05 21.72,19.05 21.72,15.24 20.7,15.24 19.05,20.32 20.32,21.59 15.88,27.3 12.06,28.57 12.06,29.84
  pour Top (isolate 0.178, rank 2): 0,0 25.4,0 25.4,82.55 0,82.55
  pour Route2 (isolate 0.178, rank 2): 0,0 25.4,0 25.4,82.55 0,82.55
  pour Bottom (isolate 0.178): 25.4,0 0,0 0,82.55 25.4,82.55
I2S_CLK_18  (via drill 0.3)
  Top 0.254: U1.36 21.04,49.45 v21.59,48.9 | IC3.5 10.1,11.76 v9.78,11.43
  Bottom 0.254: v21.59,48.9 19.68,46.99 19.68,24.77 9.78,14.86 v9.78,11.43
I2S_CLK_33
  Top 0.254: J2.3 2.54,11.43 2.87,11.76 IC3.12
I2S_RXA_18  (via drill 0.3)
  Top 0.254: U1.37 21.2,50.55 v21.59,50.16 | IC3.6 9.48,12.4 v9.14,12.06
  Bottom 0.254: v21.59,50.16 19.05,47.62 19.05,25.4 9.14,15.49 v9.14,12.06
I2S_RXA_33
  Top 0.254: IC3.11 2.83,12.4 J2.4
I2S_TXA_18  (via drill 0.3)
  Top 0.254: U1.35 20.86,48.35 v21.59,47.62 | IC3.4 10.72,11.11 v10.41,10.79
  Bottom 0.254: v21.59,47.62 20.32,46.35 20.32,24.13 10.41,14.22 v10.41,10.79
I2S_TXA_33
  Top 0.254: IC3.13 3.48,11.11 J2.2
I2S_WA_18  (via drill 0.3)
  Top 0.254: U1.34 20.7,47.25 v21.59,46.35 | IC3.3 11.34,10.46 v11.05,10.16
  Bottom 0.254: v21.59,46.35 20.95,45.72 20.95,23.5 11.05,13.59 v11.05,10.16
I2S_WA_33
  Top 0.254: IC3.14 5.38,10.46 J2.1
IO1_18  (via drill 0.3)
  Top 0.254: U1.16 4.23,51.65 v3.81,52.07
  Bottom 0.254: v3.81,52.07 3.17,51.44 3.17,47.62 TP11.1
IO2_18  (via drill 0.3)
  Top 0.254: U1.23 8.3,44.7 7.41,43.81 5.71,43.81 v5.08,44.45
  Bottom 0.254: TP12.1 v5.08,44.45
IO3_18  (via drill 0.3)
  Top 0.254: U1.24 9.4,44.71 7.87,43.18 v5.08,43.18
  Bottom 0.254: TP13.1 v5.08,43.18
IO4_18  (via drill 0.3)
  Top 0.254: U1.25 10.5,43.6 v10.92,43.18
  Bottom 0.254: TP17.1 10.92,42.42 v10.92,43.18
IO6_18  (via drill 0.3)
  Top 0.254: U1.19 3.9,48.35 v3.81,48.26
  Bottom 0.254: TP14.1 5.08,48.26 v3.81,48.26
N$1
  Top 0.254: R3.2 D5.C
N$2  (via drill 0.3)
  Top 0.254: D5.A v11.43,25.64 v11.43,25.65
  Bottom 0.254: PWR_LED.1 11.81,26.04 v11.43,25.65
N$3  (via drill 0.3)
  Top 0.254: D6.A 11.43,23.74 v11.43,23.75
  Bottom 0.254: v11.43,23.75 11.43,23.11 11.68,22.86 ON_LED.1
N$4
  Top 0.254: R4.2 D6.C
N$5  (via drill 0.3)
  Top 0.254: v2.54,37.47 D10.C
  Bottom 0.254: J2.11 2.54,33.02 v2.54,37.47
N$6
  Top 0.254: J2.12 D9.C
N$7
  Top 0.305: U2.8 18.67,16.17 R2.2
  pour Top (isolate 0.178): 16.76,14.35 18.8,14.35 19.94,15.49 19.94,16.51 16.76,16.51
N$8  (via drill 0.3)
  Top 0.254: J4.B5 14.45,5.43 v13.97,4.95 | R5.2 18,3.39 v17.78,3.17
  Bottom 0.254: v17.78,3.17 15.75,3.17 v13.97,4.95
N$9  (via drill 0.3)
  Top 0.254: J4.A5 11.45,4.97 v11.43,4.95 | R6.2 7.41,3.39 v7.62,3.17
  Bottom 0.254: v7.62,3.17 9.65,3.17 v11.43,4.95
N$10
  Top 0.239: J4.A6 12.45,6.56 12.7,6.81 13.45,6.81 | 13.45,6.81 J4.B6 | D1.3 15.74,9.91 15.89,9.76 15.89,9.29 13.45,6.85 13.45,6.81
N$11
  Top 0.239: J4.A7 12.95,5.46 12.7,5.21 12.19,5.21 11.95,5.45 J4.B7 11.95,6.67 12.52,7.24 13.23,7.24 14.59,8.59 14.59,9.76 14.74,9.91 D1.1
RI/CTS2_18  (via drill 0.3)
  Top 0.254: U1.7 4.49,61.55 v3.81,62.23
  Bottom 0.254: TP6.1 v3.81,62.23
RTS_18  (via drill 0.3)
  Top 0.254: U1.10 3.98,58.25 v3.81,58.42 | IC1.6 11.72,20.02 v11.43,20.32
  Bottom 0.254: v3.81,58.42 10.16,52.07 10.16,21.59 v11.43,20.32
RTS_33
  Top 0.254: IC1.11 5.38,20.02 4.45,20.95 4.45,26.04 J2.10 3.81,31.75 3.81,35.34 R7.2
RXD_18  (via drill 0.3)
  Top 0.254: U1.13 4.15,54.95 v3.81,54.61 | IC1.3 9.87,18.07 v9.53,18.41
  Bottom 0.254: v3.81,54.61 8.26,50.16 8.26,19.68 v9.53,18.41
RXD_33
  Top 0.254: IC1.14 3.52,18.07 2.54,19.05 2.54,20.32 J2.7
SCL_18  (via drill 0.3)
  Top 0.254: U1.27 v12.7,43.81
  Bottom 0.254: TP2.1 13.34,43.81 v12.7,43.81
SDA_18  (via drill 0.3)
  Top 0.254: U1.26 11.6,43.65 v12.06,43.18
  Bottom 0.254: TP1.1 12.06,43.81 v12.06,43.18
SHLD
  Bottom 0.254: SHLD.2 17,1.27 J4.SHLD4
  pour Route2 (isolate 0.178): 8.38,1.14 17.02,1.14 17.02,5.59 8.38,5.59
SIM_CLK  (via drill 0.3)
  Top 0.254: U1.38 21.38,51.65 v21.59,51.44 | C2.1 8.6,26.67 10.12,28.2 J1.C3 11.18,28.2 v11.43,27.94 | D4.4 18.3,39.49 v18.41,39.37
  Bottom 0.254: v11.43,27.94 12.7,27.94 18.41,33.66 v18.41,39.37 18.41,48.26 v21.59,51.44
SIM_DET  (via drill 0.3)
  Top 0.254: v11.43,35.56 11.37,35.49 J1.CD 9.17,35.49 R1.1 | U1.42 21.12,56.05 v21.59,56.52
  Bottom 0.254: v11.43,35.56 13.97,35.56 15.88,37.47 15.88,50.8 v21.59,56.52
SIM_IO  (via drill 0.3)
  Top 0.254: U1.39 21.55,52.75 v21.59,52.7 | C3.1 8.62,28.57 9.51,29.46 J1.C7 11.18,29.46 v11.43,29.21 | D4.6 18.3,42.66 v17.78,43.18
  Bottom 0.254: v11.43,29.21 12.7,29.21 17.78,34.29 v17.78,43.18 17.78,48.9 v21.59,52.7
SIM_RST  (via drill 0.3)
  Top 0.254: C1.1 8.72,30.73 J1.C2 11.18,30.73 v11.43,30.48 | U1.40 21.46,53.85 v21.59,53.98 | D4.3 16.19,40.33 v17.14,39.37
  Bottom 0.254: v11.43,30.48 12.7,30.48 17.14,34.92 v17.14,39.37 17.14,49.53 v21.59,53.98
TXD_18  (via drill 0.3)
  Top 0.254: U1.12 3.98,56.05 v3.81,55.88 | IC1.4 10.48,18.73 v10.16,19.05
  Bottom 0.254: v3.81,55.88 8.89,50.8 8.89,20.32 v10.16,19.05
TXD_33
  Top 0.254: IC1.13 4.13,18.73 3.17,19.68 3.17,22.23 J2.8
USB_N
  Top 0.239: D1.6 14.74,11.61 14.59,11.76 14.59,12.34 15.03,12.78 15.03,25.02 18.41,28.4 18.41,35.31 14.09,39.63 14.09,44.91 U1.28
USB_P
  Top 0.239: D1.4 15.74,11.61 15.89,11.76 15.89,12.34 15.45,12.78 15.45,24.85 18.83,28.23 18.83,35.48 14.52,39.8 14.52,44.46 14.62,44.56 14.62,44.92 U1.29
V_USB  (via drill 0.3)
  Top 0.239: D1.5 v15.24,12.06
  Top 0.254: U1.17 4.06,50.55 v3.81,50.8
  Top 0.508: J4.VBUS2 15.15,6.52 14.99,6.68 v14.99,7.26 14.99,7.39 15.47,7.87 16.38,7.87 16.87,7.39 F1.1
  Bottom 0.254: v3.81,50.8 6.35,50.8 7.62,49.53 7.62,10.16 10.16,7.62 14.61,7.62 | 14.61,7.62 14.61,11.43 v15.24,12.06 | v14.99,7.26 14.96,7.26 14.61,7.62
  pour Top (isolate 0.178, no thermals): 10.03,6.35 10.03,4.95 11.05,3.94 14.35,3.94 15.37,4.95 15.37,6.35
VIN
  Top 0.508: D8.A 19.43,12.19 22.73,8.89 J3.2
VSIM  (via drill 0.3)
  Top 0.254: U1.41 21.3,54.95 v21.59,55.24 | v11.43,33.02 11.18,33.27 J1.C1 9.36,33.27 C4.1 C5.1 | D4.1 15.99,42.66 v16.51,43.18
  Bottom 0.254: v11.43,33.02 12.7,33.02 16.51,36.83 v16.51,43.18 16.51,50.16 v21.59,55.24

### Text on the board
Top: 1
Route2: 2
Route15: 3
Bottom: 4 | v11
Measures: Units: inches
tDocu: 4-layer / JLC7628 Stackup / Material: TG155 / 1oz outer layers / 0.5oz inner layers / Board thickness: 1.6mm / Soldermask: Red / Silkscreen: White / Surface Finish: Lead-Free HASL | Dryw Wade

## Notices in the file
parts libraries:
SparkFun-Connectors: Licensing: Creative Commons ShareAlike 4.0 International - https://creativecommons.org/licenses/by-sa/4.0
SparkFun-Aesthetics: Released under the Creative Commons Attribution Share-Alike 4.0 License
SparkFun-Aesthetics: https://creativecommons.org/licenses/by-sa/4.0
